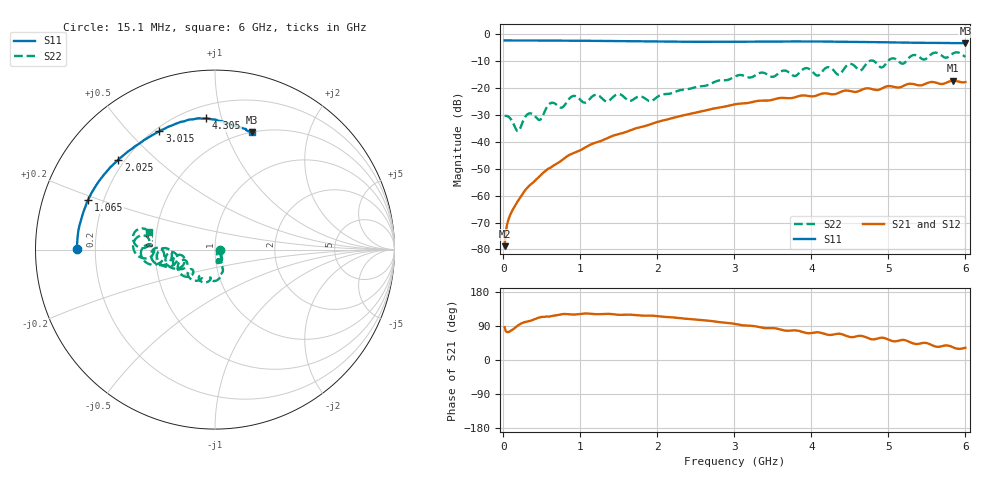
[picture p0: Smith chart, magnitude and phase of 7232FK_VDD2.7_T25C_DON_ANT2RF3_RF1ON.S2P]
!Agilent Technologies,E5071C,MY46417908,A.11.23
!Date: Fri Mar 03 11:31:44 2017
!Data & Calibration Information:
!Freq	S11:SOLT2(ON)	S21:SOLT2(ON)	S12:SOLT2(ON)	S22:SOLT2(ON)
!PortZ  Port1:50+j0  Port2:50+j0
!Above PortZ is port z conversion or system Z0 setting when saving the data.
!When reading, reference impedance value at option line is always used.
# Hz S dB R 50
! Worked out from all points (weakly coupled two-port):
!   400 points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, 15.1 MHz to 6 GHz, reference 50 ohm
!   highest |S21| = -17.25 dB at 5.835 GHz (marker M1); lowest = -78.8 dB at 15.1 MHz (marker M2)
!   lowest |S11| = -3.3 dB at 6 GHz (marker M3), VSWR 5.34, Z = 25.2 + j61.8 ohm
!   |S11| at or under -10 dB: nowhere
!   |S22| runs from -36.0 to -6.7 dB; largest |S21 - S12| = 0.0025
!   S11 on the Smith chart (normalised r, x): 15.1 MHz: 0.13, +0.00; 1.065 GHz: 0.14, +0.18; 2.025 GHz: 0.18, +0.38; 3.015 GHz: 0.22, +0.61; 4.305 GHz: 0.28, +0.90; 6 GHz: 0.50, +1.24
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1.509975e7  -2.27 179.7  -78.78 86.8  -78.64 85.2  -30.36 -5.0
3.00995e7  -2.27 179.5  -73.69 75.8  -73.55 76.9  -30.31 -11.0
7.509875e7  -2.28 178.6  -68.09 74.3  -68.09 75.0  -30.86 -29.6
1.950968e8  -2.28 176.3  -61.69 92.1  -61.65 92.2  -35.97 -30.8
2.850952e8  -2.28 174.7  -57.88 100.3  -57.87 100.7  -30.60 -26.5
4.80092e8  -2.30 171.2  -52.51 112.9  -52.49 112.9  -31.73 -55.0
6.0009e8  -2.32 168.9  -49.76 114.4  -49.77 114.4  -25.82 -45.8
7.650872e8  -2.35 165.4  -46.68 121.0  -46.70 120.9  -27.18 -57.2
9.00085e8  -2.37 162.4  -44.29 120.0  -44.30 120.1  -22.97 -58.8
1.020083e9  -2.38 159.7  -42.77 122.1  -42.79 122.0  -24.95 -71.3
1.065082e9  -2.39 158.7  -42.03 122.9  -42.05 122.8  -25.39 -65.4
1.20008e9  -2.41 155.7  -40.24 120.8  -40.25 120.9  -22.50 -67.6
1.350078e9  -2.46 152.4  -38.62 121.8  -38.63 121.7  -24.96 -70.5
1.485075e9  -2.49 149.4  -37.17 119.4  -37.18 119.4  -22.26 -75.9
2.010066e9  -2.66 137.5  -32.50 115.4  -32.51 115.5  -23.06 -62.1
2.025066e9  -2.67 137.1  -32.38 115.1  -32.39 115.1  -22.78 -63.0
3.01505e9  -2.75 115.2  -25.98 94.8  -25.97 94.9  -15.57 -83.7
4.005033e9  -2.65 97.9  -23.07 71.3  -23.06 71.0  -13.62 -161.3
4.305028e9  -2.69 93.7  -22.25 68.1  -22.28 67.9  -13.96 -171.8
5.010016e9  -3.00 85.3  -19.22 52.9  -19.15 53.2  -9.51 -166.0
5.835003e9  -3.27 74.7  -17.25 33.8  -17.20 34.8  -7.16 177.2
6e9  -3.29 72.4  -17.74 32.2  -17.77 33.1  -8.38 165.2
